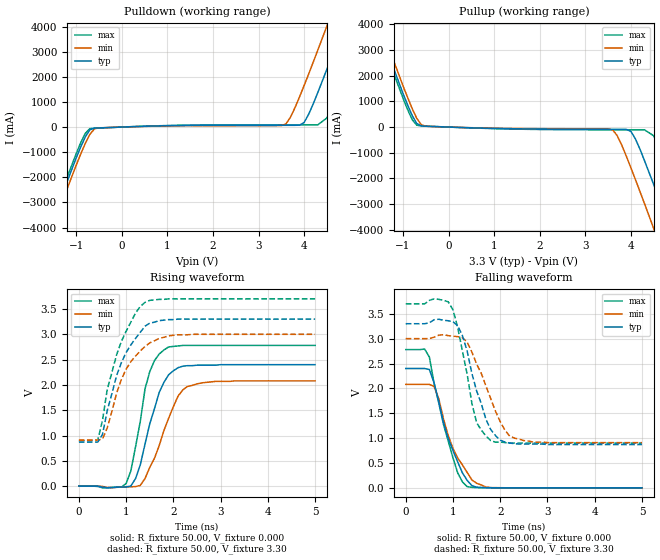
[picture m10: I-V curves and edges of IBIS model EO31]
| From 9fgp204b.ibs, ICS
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|   Model EO31
[Model]   EO31
Model_type   Output
Polarity   Non-Inverting
Vmeas =   1.50V
Cref =  30.00pF
Rref =  83.000
Vref =   1.50V
C_comp   3.40pF   2.85pF   3.95pF
[Temperature Range]   27.00   70.00   0.000
[Voltage Range]   3.30V   3.00V   3.70V
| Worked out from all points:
|   slope of the pulldown table from 0 to 0.495 V, typ, clamps not added: 16 ohm
|   slope of the pullup table from 0 to 0.495 V, typ, clamps not added: 17.2 ohm
|   rising waveform, R_fixture 50.00, V_fixture 0.000: 20-80 % time 420ps typ, 519ps min, 336ps max; typ from 0 V to 2.4 V
|   rising waveform, R_fixture 50.00, V_fixture 3.30: 20-80 % time 547ps typ, 558ps min, 518ps max; typ from 0.87 V to 3.3 V
|   falling waveform, R_fixture 50.00, V_fixture 0.000: 20-80 % time 468ps typ, 499ps min, 438ps max; typ from 2.4 V to 0 V
|   falling waveform, R_fixture 50.00, V_fixture 3.30: 20-80 % time 428ps typ, 540ps min, 345ps max; typ from 3.3 V to 0.87 V
[Pulldown]
| voltage   I(typ)   I(min)   I(max)
-3.3V     -12.43A    -12.7A     -12.26A
-1.7V     -4.56A     -4.85A     -4.38A
-1.5V     -3.59A     -3.88A     -3.41A
-900mV    -790mA     -1.07A     -620mA
-700mV    -110mA     -290mA     -63.37mA
3.6V      70.03mA    120mA      86.32mA
4V        180mA      1.65A      86.59mA
4.3V      1.37A      3.06A      87.5mA
4.5V      2.3A       4.02A      360mA
4.9V      4.22A      5.96A      2.13A
5.3V      6.17A      7.92A      4.05A
6.6V      12.6A      14.35A     10.47A
[Pullup]
| voltage   I(typ)   I(min)   I(max)
-3.3V     12.5A      12.79A     12.33A
-1.7V     4.63A      4.93A      4.45A
-1.5V     3.67A      3.96A      3.48A
-700mV    140mA      340mA      72.8mA
-500mV    33.12mA    32.35mA    36.23mA
3.6V      -85.44mA   -110mA     -110mA
4V        -170mA     -1.59A     -110mA
4.3V      -1.32A     -2.99A     -110mA
4.5V      -2.24A     -3.95A     -340mA
4.9V      -4.16A     -5.89A     -2.09A
5.3V      -6.11A     -7.85A     -4.01A
6.6V      -12.52A    -14.26A    -10.39A
[Ramp]
| variable   typ   min   max
dV/dt_r   1.44/0.41n   1.25/0.50n   1.67/0.36n
dV/dt_f   1.46/0.42n   1.26/0.51n   1.68/0.36n
R_load = 50.00
[Rising Waveform]
R_fixture = 50.00
V_fixture = 0.000
V_fixture_min = 0.000
V_fixture_max = 0.000
| time   V(typ)   V(min)   V(max)
0s        0V         0V         0V
1ns       -16.84mV   -14.71mV   51.16mV
1.2ns     150mV      -8.86mV    780mV
1.4ns     830mV      150mV      1.92V
1.5ns     1.23V      370mV      2.26V
1.7ns     1.85V      800mV      2.61V
1.9ns     2.2V       1.34V      2.75V
2.2ns     2.37V      1.9V       2.78V
2.5ns     2.39V      2.02V      2.78V
5ns       2.4V       2.08V      2.78V
[Rising Waveform]
R_fixture = 50.00
V_fixture = 3.30
V_fixture_min = 3.00
V_fixture_max = 3.70
| time   V(typ)   V(min)   V(max)
0s        870mV      910mV      900mV
400ps     870mV      910mV      910mV
500ps     1.02V      930mV      1.3V
600ps     1.49V      1.15V      1.91V
800ps     2.19V      1.84V      2.6V
1ns       2.64V      2.31V      3.06V
1.2ns     2.92V      2.57V      3.42V
1.4ns     3.16V      2.76V      3.63V
2.1ns     3.3V       2.99V      3.7V
5ns       3.3V       3V         3.7V
[Falling Waveform]
R_fixture = 50.00
V_fixture = 0.000
V_fixture_min = 0.000
V_fixture_max = 0.000
| time   V(typ)   V(min)   V(max)
0s        2.4V       2.08V      2.78V
400ps     2.4V       2.08V      2.79V
500ps     2.38V      2.08V      2.63V
600ps     2.11V      2.04V      2.1V
700ps     1.73V      1.79V      1.7V
1ns       750mV      790mV      600mV
1.1ns     520mV      600mV      300mV
1.3ns     150mV      310mV      24.88mV
1.8ns     2.02mV     5.61mV     1.06mV
5ns       -14.97uV   19.03uV    13.75uV
[Falling Waveform]
R_fixture = 50.00
V_fixture = 3.30
V_fixture_min = 3.00
V_fixture_max = 3.70
| time   V(typ)   V(min)   V(max)
0s        3.3V       3V         3.7V
900ps     3.36V      3.06V      3.74V
1ns       3.34V      3.05V      3.58V
1.2ns     3.06V      3.02V      2.75V
1.4ns     2.3V       2.73V      1.7V
1.5ns     1.95V      2.49V      1.31V
1.8ns     1.17V      1.79V      950mV
2.1ns     920mV      1.16V      910mV
2.3ns     890mV      1V         900mV
5ns       870mV      910mV      900mV
